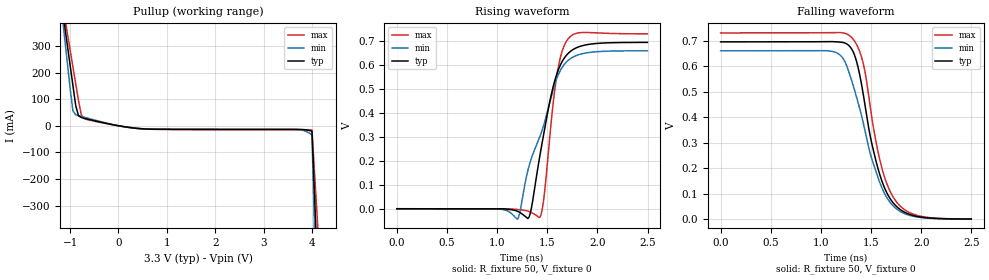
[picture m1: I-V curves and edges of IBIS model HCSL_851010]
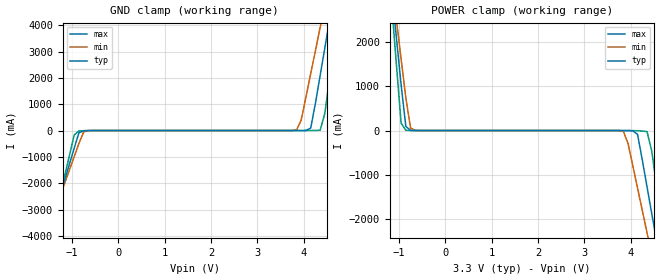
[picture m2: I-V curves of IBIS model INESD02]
|   This file is an IBIS representation of the   |
|   Integrated Device Technology , Inc.   |
|   ICS851010   |
|  1-TO-10 DIFFERENTIAL CURRENT MODE 0.7V DIFFERENTIAL HCSL FANOUT BUFFER  |
[IBIS Ver]   4.1
[File name]   851010i.ibs
[File Rev]   1.1
|v1.1 Removed "475 Rref" option, which is not used
|v1.0 Original
[Date]   Nov 12 2020 | Last modified
|   Dec 21 2006 | Generated
[Source]   Originated at Integrated Device Technology, Inc.
[Disclaimer]
IDT hereby grants the user of this IBIS model a non-exclusive,
nontransferable license to use this IBIS model under the following terms.
Before using this IBIS model, the user should read this license.
If the user does not accept these terms,  the IBIS model should be
returned to IDT within 30 days.
   The user is granted this license only to use the IBIS model and
is not granted rights to sell, load, rent, lease or license the IBIS
model in whole or in part, or in modified form to anyone other than
user. User may modify the IBIS model to suit its specific
applications but rights to derivative works and such modifications
shall belong to IDT.
   This IBIS model is provided on an "AS IS" basis and IDT makes
absolutely no warranty with respect to the information contained
herein. IDT DISCLAIMS AND CUSTOMER WAIVES ALL WARRANTIES, EXPRESS
OR IMPLIED, INCLUDING WARRANTIES OF MERCHANTABILITY OR FITNESS FOR
A PARTICULAR PURPOSE. The entire risk as to quality and performance
is with the Customer. ACCORDINGLY, IN NO EVENT SHALL THE COMPANY BE
LIABLE FOR ANY DAMAGES, WHETHER IN CONTRACT OR TORT,INCLUDING ANY
LOST PROFITS OR OTHER INCIDENTAL, CONSEQUENTIAL, EXEMPLARY, OR
PUNITIVE DAMAGES ARISING OUT OF THE USE OR APPLICATION OF THE IBIS
model provided in this package. Further, IDT reserves the right to
make changes without notice to any product herein to improve
reliability, function, or design. IDT does not convey any license
under patent rights or any other intellectual property rights,
including those of third parties.
   IDT is not obligated to provide maintenance or support
for the licensed IBIS model.
[Copyright]   Copyright 2006 by Integrated Device Technology, Inc.
[Component]   ICS851010AY
[Manufacturer] Integrated Device Technology, Inc.
[Package]
|LQFP32
|lead + wire   typ   min   max
R_pkg   220.4m   212.5m   238m
L_pkg   1.841n   1.708n   1.974n
C_pkg   0.316p   0.2907p   0.33p
[Pin] signal_name   model_name   R_pin   L_pin   C_pin
1   Q0   HCSL_851010   238m   1.974n   0.330p
2   nQ0   HCSL_851010   225m   1.841n   0.311p
3   VDD   POWER   218m   1.7745n   0.301p
4   Q1   HCSL_851010   213m   1.708n   0.291p
5   nQ1   HCSL_851010   213m   1.708n   0.291p
6   Q2   HCSL_851010   218m   1.7745n   0.301p
7   nQ2   HCSL_851010   225m   1.841n   0.311p
8   VDD   POWER   238m   1.974n   0.330p
9   GND   GND   238m   1.974n   0.330p
10   IREF   NC   225m   1.841n   0.311p
11   Q3   HCSL_851010   218m   1.7745n   0.301p
12   nQ3   HCSL_851010   213m   1.708n   0.291p
13   VDD   POWER   213m   1.708n   0.291p
14   VDD   POWER   218m   1.7745n   0.301p
15   Q4   HCSL_851010   225m   1.841n   0.311p
16   nQ4   HCSL_851010   238m   1.974n   0.330p
17   VDD   POWER   238m   1.974n   0.330p
18   Q5   HCSL_851010   225m   1.841n   0.311p
19   nQ5   HCSL_851010   218m   1.7745n   0.301p
20   Q6   HCSL_851010   213m   1.708n   0.291p
21   nQ6   HCSL_851010   213m   1.708n   0.291p
22   VDD   POWER   218m   1.7745n   0.301p
23   Q7   HCSL_851010   225m   1.841n   0.311p
24   nQ7   HCSL_851010   238m   1.974n   0.330p
25   GND   GND   238m   1.974n   0.330p
26   CLK   INESD02   225m   1.841n   0.311p
27   nCLK   INESD02   218m   1.7745n   0.301p
28   Q8   HCSL_851010   213m   1.708n   0.291p
29   nQ8   HCSL_851010   213m   1.708n   0.291p
30   VDD   POWER   218m   1.7745n   0.301p
31   Q9   HCSL_851010   225m   1.841n   0.311p
32   nQ9   HCSL_851010   238m   1.974n   0.330p
[Diff Pin]  inv_pin  vdiff tdelay_typ tdelay_min  tdelay_max
|Input
26   27   0.15   0   0   0
|Outputs
1   2   NA   0   0   0
4   5   NA   0   0   0
6   7   NA   0   0   0
11   12   NA   0   0   0
15   16   NA   0   0   0
18   19   NA   0   0   0
20   21   NA   0   0   0
23   24   NA   0   0   0
28   29   NA   0   0   0
31   32   NA   0   0   0
| Models and submodels in the file (2): HCSL_851010 (Open_source), INESD02 (Input)
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[Model]   HCSL_851010
Model_type   Open_source
Polarity   Non-Inverting
|   typ   min   max
C_comp   2pF   1.5pF   2.5pF
Vmeas = 0.345V
Rref= 50
Cref = 0
Vref = 0V
|   typ   min   max
[Voltage range]   3.3V   3.135V   3.465V
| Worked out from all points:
|   slope of the pullup table from 0 to 0.495 V, typ, clamps not added: 43.2 ohm
|   rising waveform, R_fixture 50, V_fixture 0: 20-80 % time 196ps typ, 289ps min, 115ps max; typ from 0 V to 0.696 V
|   falling waveform, R_fixture 50, V_fixture 0: 20-80 % time 225ps typ, 279ps min, 214ps max; typ from 0.696 V to 0 V
[Pullup]
|Voltage   I (typ)   I (min)   I (max)
-3.3V     3.285A     4.012A     2.855A
-1.46V    833.2mA    911mA      792.2mA
-1V       227.7mA    140.2mA    285.3mA
-941.5mV  150.8mA    55.31mA    221.1mA
-884.1mV  75.28mA    41.59mA    158mA
-826.6mV  37.56mA    38.03mA    94.9mA
-769.2mV  31.15mA    35.07mA    41.37mA
-654.2mV  25.62mA    29.28mA    23.51mA
552.4mV   -12.05mA   -12.01mA   -11.89mA
4.001V    -20.76mA   -34.36mA   -15.97mA
4.521V    -2.384A    -3.623A    -1.596A
6.6V      -15.32A    -20.11A    -12.39A
[Ramp]
|   typ   min   max
dV/dt_r   0.588/0.302n   0.562/0.4n   0.619/0.183n
dV/dt_f   0.557/0.358n   0.529/0.424n   0.585/0.357n
R_load =   50.0000
[Rising Waveform]
R_fixture = 50
V_fixture = 0   | VCC_typ
V_fixture_max = 0   | VCC_max
V_fixture_min = 0   | VCC_min
C_fixture = 0.0p
| Time   typ   min   max
0s        161.4pV    155.5pV    177.6pV
1.004ns   257.4uV    -345.7uV   171.5uV
1.204ns   -10.7mV    -42.63mV   -3.041mV
1.321ns   -31.32mV   183.8mV    -12.21mV
1.424ns   217.1mV    299.1mV    -35.81mV
1.466ns   318.2mV    352.6mV    46.44mV
1.589ns   556.2mV    539.5mV    542.4mV
1.689ns   641.1mV    613.2mV    699.5mV
1.829ns   679.4mV    646.3mV    736.3mV
2.498ns   695.6mV    660.5mV    731.1mV
[Falling Waveform]
R_fixture = 50
V_fixture = 0   | VCC_typ
V_fixture_max = 0   | VCC_max
V_fixture_min = 0   | VCC_min
C_fixture = 0.0p
| Time   typ   min   max
0s        695.7mV    660.7mV    730.9mV
1.109ns   696.7mV    658.7mV    732.5mV
1.284ns   679mV      571.8mV    720.6mV
1.349ns   627.2mV    487.1mV    689.9mV
1.411ns   513.6mV    394.7mV    626.2mV
1.494ns   319.9mV    253.1mV    431.8mV
1.584ns   177.3mV    145.9mV    236.6mV
1.732ns   58.14mV    47.13mV    78.96mV
1.964ns   9.932mV    7.789mV    13.86mV
2.498ns   174uV      126.1uV    260.7uV
[Model]   INESD02
Model_type   Input
Polarity   Non-Inverting
Vinl = 1.10V
Vinh = 2.2V
|   typ   min   max
C_comp   2pF   1.5pF   2.5pF
|   typ   min   max
[Voltage range]  3.3V   3.15V   3.45V
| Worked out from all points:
|   GND clamp passes 1 mA (typ) near -0.58 V on its own axis
|   POWER clamp passes 1 mA (typ) near -0.68 V on its own axis
[GND_clamp]
|Voltage   I(typ)   I(min)   I(max)
-3.3V     -14.52A    -12.53A    -17.87A
-1.565V   -4.277A    -3.994A    -4.784A
-1.463V   -3.675A    -3.492A    -4.014A
-952.6mV  -663.4mA   -987.4mA   -164.5mA
-850.5mV  -87.58mA   -487.5mA   -16.02mA
-646.4mV  -1.897mA   -2.647mA   -4.136mA
3.844V    27.46uA    16.34mA    91.61nA
4.151V    91.22mA    2.153A     394uA
4.355V    2.088A     3.911A     12mA
4.559V    4.201A     5.67A      2.008A
4.763V    6.316A     7.429A     4.712A
6.6V      25.37A     23.29A     29.07A
[POWER_clamp]
|Voltage   I(typ)   I(min)   I(max)
-3.3V     25.37A     21.86A     31.26A
-1.157V   3.144A     3.369A     2.841A
-1.055V   2.088A     2.49A      1.49A
-952.6mV  1.032A     1.611A     167.9mA
-850.5mV  91.22mA    733.4mA    4.648mA
-646.4mV  248.7uA    2.242mA    177.6uA
3.844V    -406.9uA   -15.83mA   -19.94uA
4.151V    -87.58mA   -1.296A    -5.896mA
4.355V    -1.265A    -2.297A    -23.82mA
4.559V    -2.47A     -3.3A      -1.229A
4.763V    -3.675A    -4.303A    -2.769A
6.6V      -14.52A    -13.34A    -16.62A
